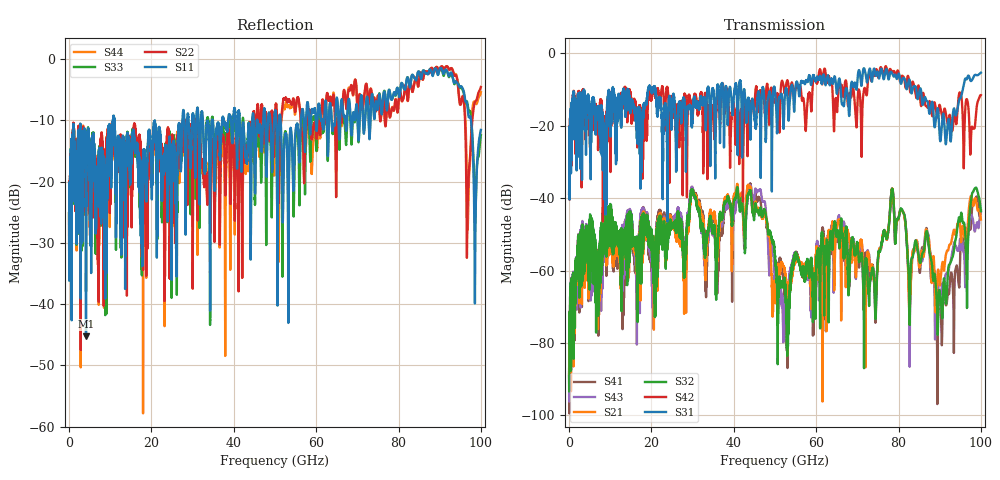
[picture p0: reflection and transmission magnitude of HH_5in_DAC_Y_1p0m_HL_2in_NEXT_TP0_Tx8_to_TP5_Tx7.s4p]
# GHz S RI R 45
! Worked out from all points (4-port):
!   4000 points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, 25 MHz to 100 GHz, reference 45 ohm
!   strongest paths, dB at 25 MHz, 25.02 GHz, 50.02 GHz, 75.03 GHz, 100 GHz:
!     S31: -38.8, -15.8, -10.6, -5.5, -5.3
!     S42: -38.8, -15.0, -12.9, -6.4, -11.5
!     S32: -89.2, -47.0, -55.9, -56.5, -43.6
!     S21: -88.8, -47.2, -63.8, -57.5, -45.9
!     S43: -87.2, -46.4, -64.4, -57.5, -43.6
!     S41: -88.1, -45.6, -57.7, -56.4, -43.4
!   lowest |S11| = -45.2 dB at 4.125 GHz (marker M1), VSWR 1.01, Z = 45.3 + j0.381 ohm
!   |S11| at or under -10 dB: start of sweep to 10.65 GHz; 11.01 GHz to 20.85 GHz (9.842 GHz wide, 61.8 % of centre); 20.85 GHz to 27.52 GHz (6.667 GHz wide, 27.6 % of centre)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
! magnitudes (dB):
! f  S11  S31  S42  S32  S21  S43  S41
! 25 MHz  -25.2  -38.8  -38.8  -89.2  -88.8  -87.2  -88.1
! 4.125 GHz  -45.2  -28.0  -22.9  -50.6  -53.1  -49.3  -51.7
! 46.15 GHz  -11.7  -11.2  -13.1  -44.8  -43.9  -38.0  -40.1
! 52.4 GHz  -12.8  -11.8  -10.9  -63.0  -60.7  -66.9  -66.7
! 78.42 GHz  -6.6  -5.5  -5.1  -37.4  -37.3  -37.4  -37.4
! 90.38 GHz  -1.5  -22.0  -16.3  -69.5  -60.3  -65.5  -74.5
! 100 GHz  -11.5  -5.3  -11.5  -43.6  -45.9  -43.6  -43.4
